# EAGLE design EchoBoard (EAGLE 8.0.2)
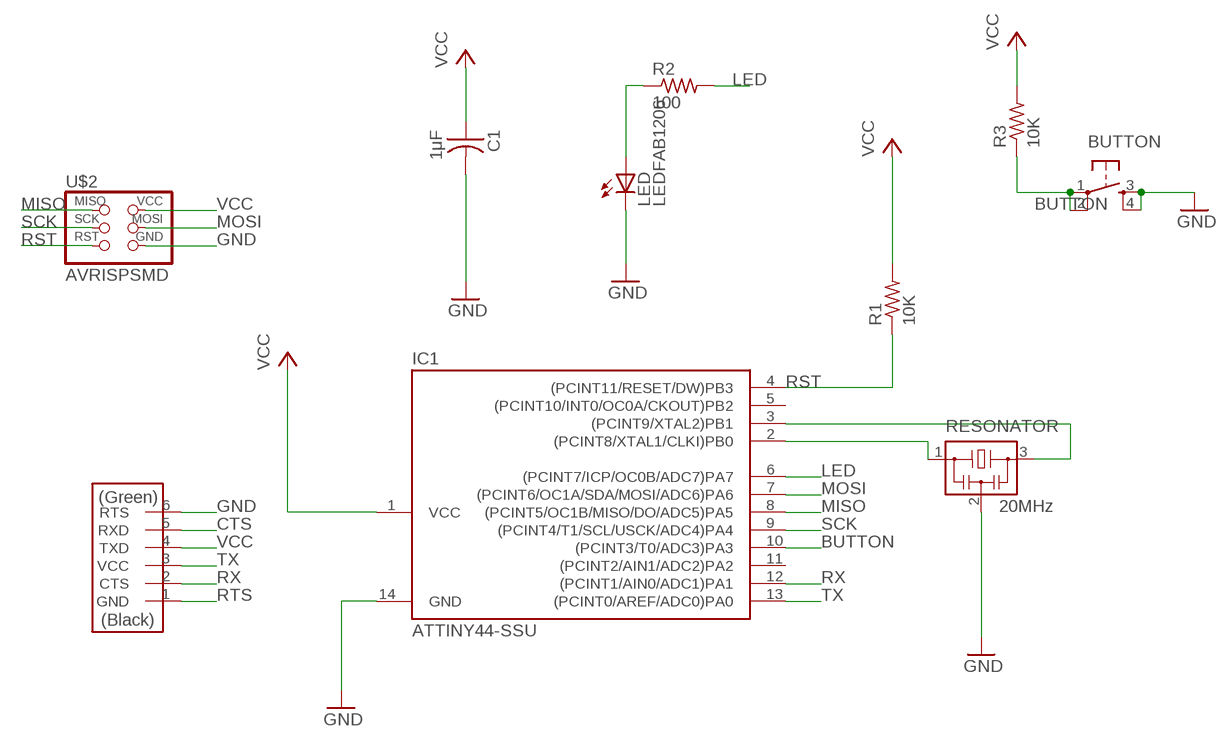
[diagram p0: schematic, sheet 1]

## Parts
BUTTON  6MM_SWITCH6MM_SWITCH  [6MM_SWITCH]
C1  1μF  CAP-US1206FAB  [C1206FAB]
IC1  ATTINY44-SSU  [SOIC14]
LED  LEDFAB1206  [LED1206FAB]
R1  10K  RES-US1206FAB  [R1206FAB]
R2  100  RES-US1206FAB  [R1206FAB]
R3  10K  RES-US1206FAB  [R1206FAB]
RESONATOR  20MHz  RESONATOR  [EFOBM]
U$2  AVRISPSMD  [2X03SMD]
U$3  FTDI-SMD-HEADER  [1X06SMD]

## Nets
BUTTON: BUTTON.1(P) BUTTON.2(P1) IC1.10((PCINT3/T0/ADC3)PA3) R3.1
CTS: U$3.5(RXD)
GND: BUTTON.3(S) BUTTON.4(S1) C1.2 IC1.14(GND) LED.2(C) RESONATOR.2 U$2.6(GND) U$3.6(RTS)
LED: IC1.6((PCINT7/ICP/OC0B/ADC7)PA7) R2.2
MISO: IC1.8((PCINT5/OC1B/MISO/DO/ADC5)PA5) U$2.1(MISO)
MOSI: IC1.7((PCINT6/OC1A/SDA/MOSI/ADC6)PA6) U$2.4(MOSI)
N$1: LED.1(A) R2.1
N$4: IC1.3((PCINT9/XTAL2)PB1) RESONATOR.3
N$5: IC1.2((PCINT8/XTAL1/CLKI)PB0) RESONATOR.1
RST: IC1.4((PCINT11/RESET/DW)PB3) R1.1 U$2.5(RST)
RTS: U$3.1(GND)
RX: IC1.12((PCINT1/AIN0/ADC1)PA1) U$3.2(CTS)
SCK: IC1.9((PCINT4/T1/SCL/USCK/ADC4)PA4) U$2.3(SCK)
TX: IC1.13((PCINT0/AREF/ADC0)PA0) U$3.3(VCC)
VCC: C1.1 IC1.1(VCC) R1.2 R3.2 U$2.2(VCC) U$3.4(TXD)
Unconnected: IC1.5((PCINT10/INT0/OC0A/CKOUT)PB2) IC1.11((PCINT2/AIN1/ADC2)PA2)

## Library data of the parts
BUTTON = fab:6MM_SWITCH: OMRON SWITCH
C1 = fab:CAP-US
IC1 = fab:ATTINY44
LED = fab:LED: LED
R1-R3 = fab:RES-US: Resistor (US Symbol)
RESONATOR = fab:RESONATOR
U$2 = fab:AVRISP
U$3 = fab:FTDI-SMD-HEADER

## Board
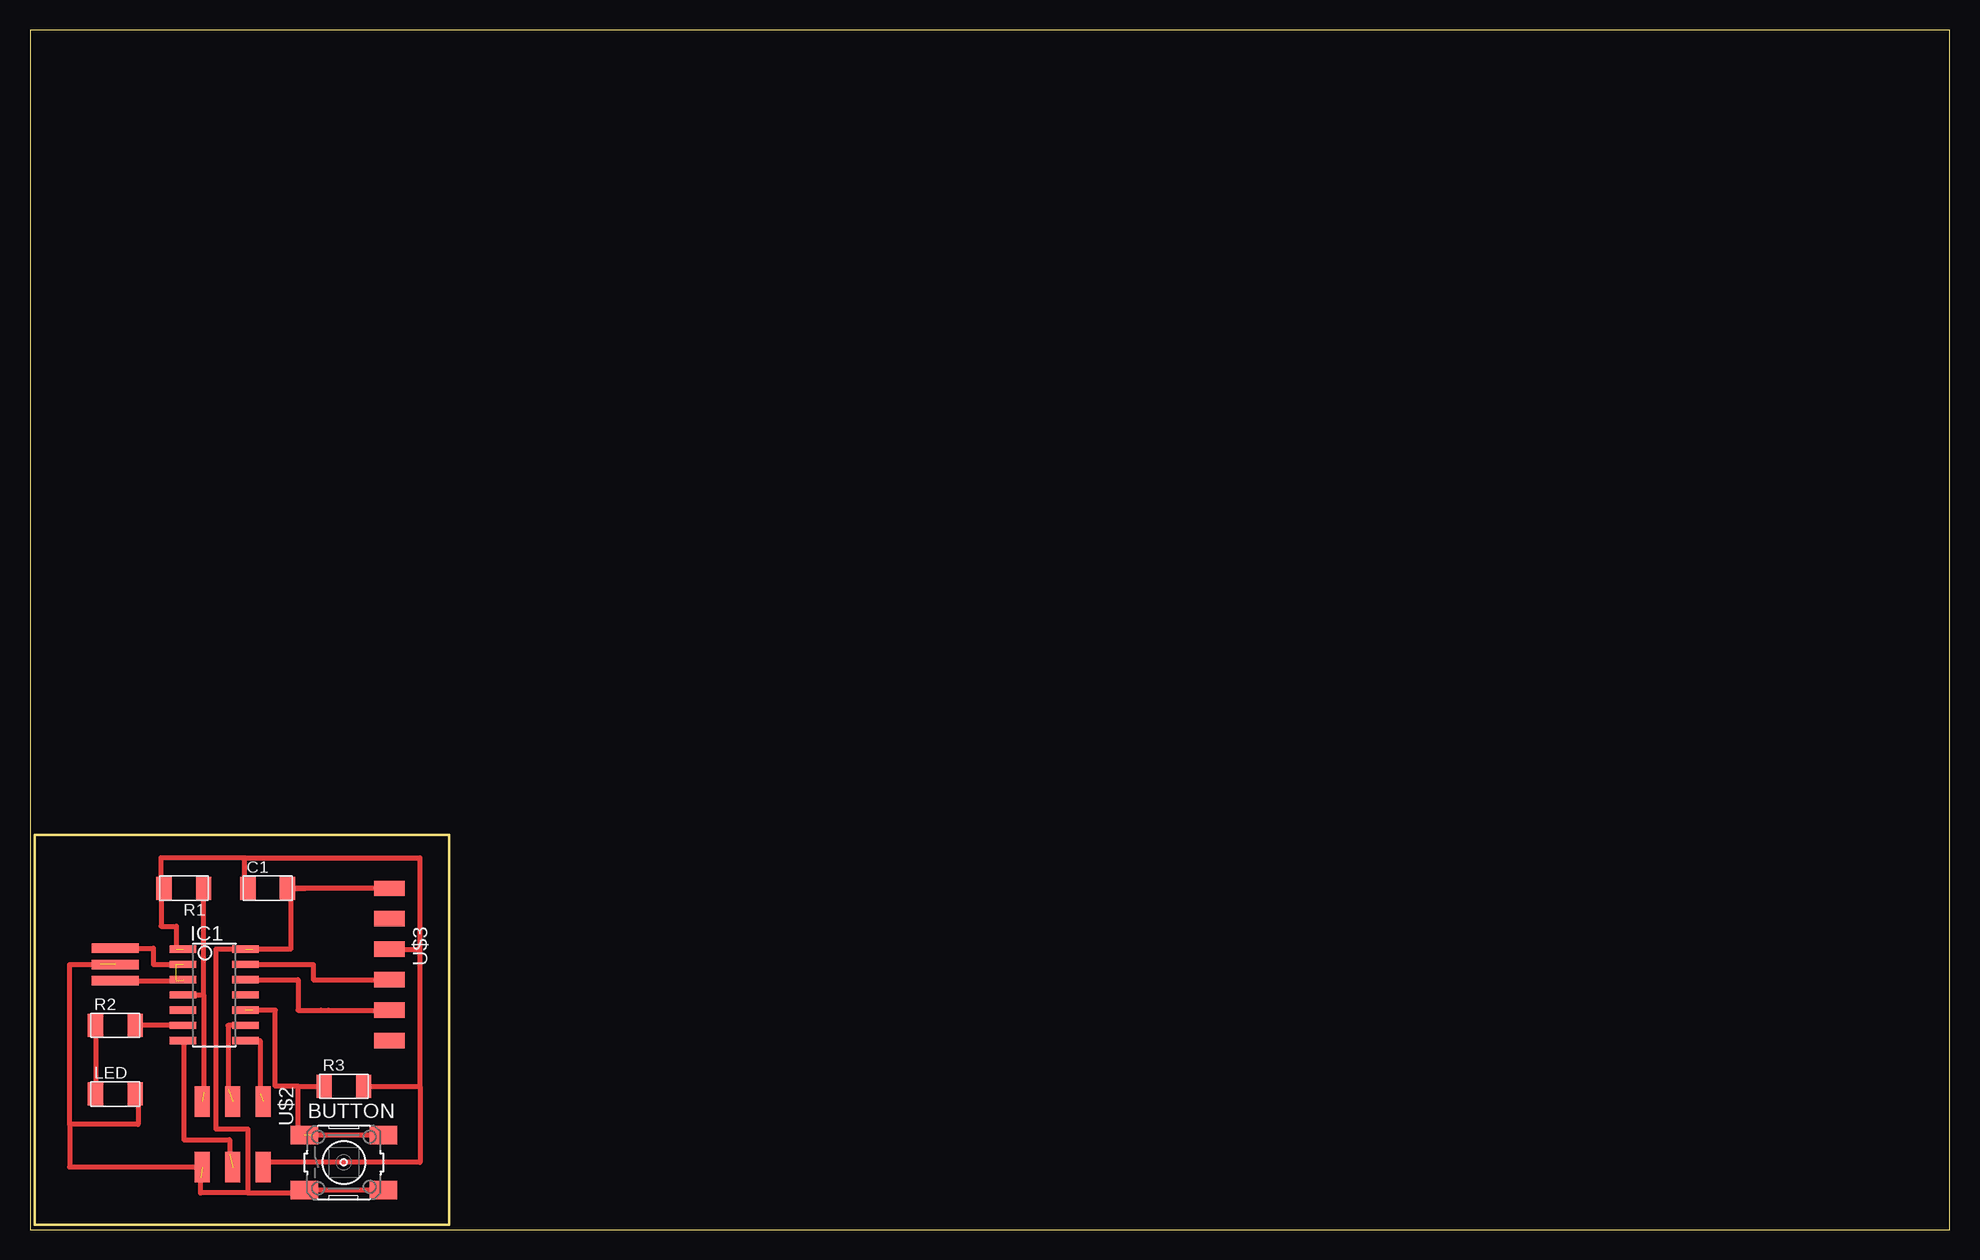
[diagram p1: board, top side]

Size 160 x 100 mm. Coordinates in mm from the lower left corner, seen from the top.
Outline: 0,0 160,0 160,100 0,100 0,0
Outline: 0.38,0.38 0.38,32.89 34.92,32.89 34.92,0.38 0.38,0.38
Copper layers (1*16): Top 0.035mm / dielectric 1.5mm / Bottom 0.035mm
Design rules "default": minimum track width 10mil, minimum drill 24mil, track to track 8mil, track to pad 8mil, pad to pad 8mil, via to via 8mil, smd to smd 8mil, copper to edge 40mil, drill to drill 8mil, minimum pad ring 10mil, minimum via ring 8mil, stop-mask expansion 4mil, vias tented up to drill 0mil, thermal gap 10mil

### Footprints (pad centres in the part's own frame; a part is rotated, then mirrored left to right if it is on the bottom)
6MM_SWITCH = smd 2.286 x 1.524: 1 -3.302,2.286; 2 3.302,2.286; 3 -3.302,-2.286; 4 3.302,-2.286
C1206FAB = smd 1.27 x 1.905: 1 -1.651,0; 2 1.651,0
SOIC14 = smd 0.61 x 2.21: 1 -3.81,-2.603; 2 -2.54,-2.603; 3 -1.27,-2.603; 4 0,-2.603; 5 1.27,-2.603; 6 2.54,-2.603; 7 3.81,-2.603; 8 3.81,2.603; 9 2.54,2.603; 10 1.27,2.603; 11 0,2.603; 12 -1.27,2.603; 13 -2.54,2.603; 14 -3.81,2.603
LED1206FAB = smd 1.27 x 1.905: 1 -1.651,0; 2 1.651,0
R1206FAB = smd 1.27 x 1.905: 1 -1.651,0; 2 1.651,0
EFOBM = smd 0.8 x 3.9: 1 -1.35,0; 2 0,0; 3 1.35,0
2X03SMD = smd 2.54 x 1.27: 1 -2.54,2.54; 2 2.92,2.54; 3 -2.54,0; 4 2.92,0; 5 -2.54,-2.54; 6 2.92,-2.54
1X06SMD = smd 2.54 x 1.27: 1 0,6.35; 2 0,3.81; 3 0,1.27; 4 0,-1.27; 5 0,-3.81; 6 0,-6.35

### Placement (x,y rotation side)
BUTTON  26.16,5.59 0 top
C1  19.81,28.45 0 top
IC1  15.37,19.56 270 top
LED  7.11,11.3 0 top
R1  12.83,28.45 180 top
R2  7.11,17.02 0 top
R3  26.16,11.94 0 top
RESONATOR  7.11,22.1 270 top
U$2  16.89,8.13 270 top
U$3  29.97,22.1 180 top

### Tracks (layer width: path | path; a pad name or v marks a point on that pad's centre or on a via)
BUTTON  (2 unrouted)
  Top 0.406: BUTTON.2 23.62,7.87 23.62,7.49 | 18.54,18.29 20.45,18.29 20.45,11.94 22.35,11.94 | 22.35,11.94 R3.1 | BUTTON.1 22.35,7.87 22.35,11.94
GND  (3 unrouted)
  Top 0.406: U$3.6 C1.2 | U$2.6 3.3,5.21 3.3,8.76 | 3.3,8.76 3.3,22.1 5.84,22.1 | LED.2 9.02,11.3 9.02,8.76 3.3,8.76 | 23.37,3.3 BUTTON.4 | 23.37,3.3 BUTTON.3 | C1.2 22.99,28.45 | C1.2 21.72,28.45 21.72,23.37 18.54,23.37 | IC1.14 15.49,23.37 15.49,8.38 18.16,8.38 18.16,3.05 | 14.22,4.32 14.22,3.05 18.16,3.05 | 18.16,3.05 23.37,3.05 23.37,3.3
LED
  Top 0.406: IC1.6 R2.2
MISO  (1 unrouted)
  Top 0.406: 18.54,15.75 IC1.8 19.18,15.75 19.18,11.3
MOSI  (1 unrouted)
  Top 0.406: IC1.7 12.83,15.75 12.83,7.49 16.64,7.49 16.64,6.22
N$1
  Top 0.406: R2.1 LED.1
N$4  (1 unrouted)
  Top 0.406: RESONATOR.3 12.19,20.75 12.19,20.83
N$5  (2 unrouted)
  Top 0.406: 12.19,20.75 12.19,20.83 | RESONATOR.1 10.29,23.45 10.29,22.1 12.19,22.1
RST  (1 unrouted)
  Top 0.406: 14.48,19.56 R1.1 | 14.48,19.56 14.48,11.43 | IC1.4 14.48,19.56
RX
  Top 0.406: IC1.12 22.35,20.83 22.35,18.29 24.26,18.29 24.89,18.29 U$3.2
SCK  (1 unrouted)
  Top 0.406: IC1.9 16.51,17.02 16.51,11.68
TX
  Top 0.406: IC1.13 23.62,22.1 23.62,20.83 U$3.3
VCC  (1 unrouted)
  Top 0.406: 10.92,28.45 10.92,30.99 17.91,30.99 | 17.91,30.99 32.51,30.99 32.51,23.37 | 32.51,11.94 32.51,23.37 | 32.51,11.94 32.51,5.59 19.18,5.59 U$2.2 | U$3.4 32.51,23.37 | C1.1 17.91,28.45 17.91,30.99 | R3.2 32.51,11.94 | R1.2 10.92,28.45 | 10.92,28.45 10.92,25.27 12.19,25.27 12.19,23.37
